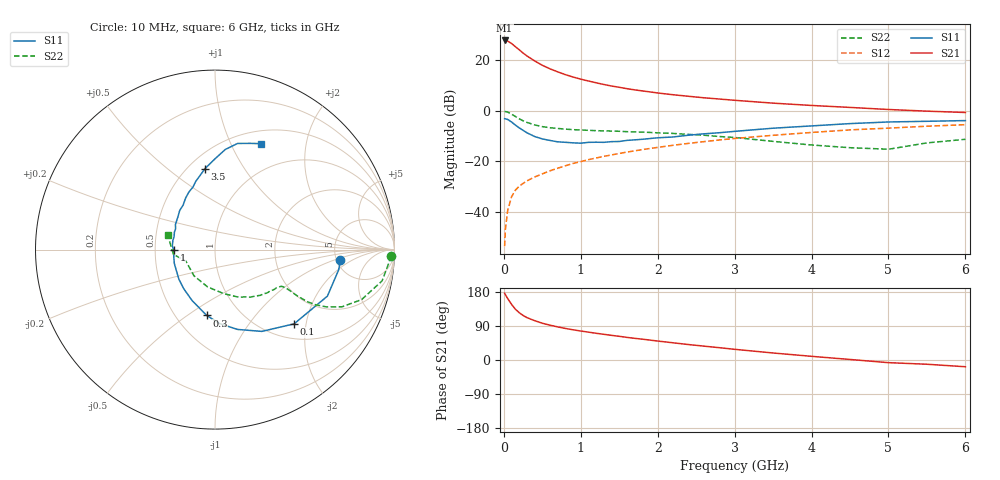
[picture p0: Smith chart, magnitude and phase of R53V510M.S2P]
! SIEMENS Small Signal Semiconductors
! BFR183
! Si NPN RF Bipolar Junction Transistor in SOT23
! VCE = 3.5 V  IC = 10 mA
! Common Emitter S-Parameters:  May  1996
# GHz  S  MA  R  50
!  f  S11  S21  S12  S22
! GHz  MAG  ANG  MAG  ANG  MAG  ANG  MAG  ANG
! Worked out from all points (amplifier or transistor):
!   36 points, 10 MHz to 6 GHz, reference 50 ohm
!   highest |S21| = 27.9 dB at 10 MHz (marker M1)
!   |S21| within 3 dB of that: start of sweep to 172 MHz
!   unconditionally stable (mu >= 1): 774.2 MHz to 2.476 GHz
!   at 250 MHz: K = 0.62, MSG = 25.8 dB, |S12| = -28.7 dB
!   at 1.4 GHz: K = 1.05, MAG = 12.2 dB, |S12| = -17.4 dB
!   at 6 GHz: K = 0.89, MSG = 2.4 dB, |S12| = -5.4 dB
!   lowest NFmin = 1.30 dB at 450 MHz
!   S11 on the Smith chart (normalised r, x): 10 MHz: 5.40, -1.25; 100 MHz: 1.31, -1.71; 300 MHz: 0.70, -0.60; 1 GHz: 0.63, -0.00; 3.5 GHz: 0.60, +0.69; 6 GHz: 0.65, +1.31
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0.01  0.7016 -4.8  24.85 176.3  0.0021 86.6  0.9796 -2.0
0.02  0.6982 -9.3  24.68 172.4  0.0045 86.1  0.972 -4.3
0.05  0.6778 -22.5  24.16 162.1  0.0107 79.8  0.947 -10.6
0.1  0.6044 -43.2  21.63 146.9  0.0199 72.1  0.8633 -18.8
0.15  0.5252 -60.2  18.73 134.0  0.027 66.0  0.7769 -24.2
0.2  0.4623 -74.2  16.25 124.8  0.0323 64.0  0.6988 -27.2
0.25  0.4132 -86.4  14 117.6  0.0367 62.8  0.6369 -28.8
0.3  0.3695 -97.2  12.28 111.9  0.0412 62.8  0.5933 -29.4
0.4  0.3116 -114.1  9.789 103.8  0.0491 62.9  0.5293 -29.4
0.5  0.2792 -128.5  8.017 97.0  0.0567 63.9  0.4884 -28.9
0.6  0.2604 -140.5  6.822 91.9  0.0652 64.6  0.4651 -28.6
0.7  0.2445 -152.0  5.936 87.4  0.0733 65.1  0.4498 -28.5
0.8  0.2393 -161.4  5.228 83.3  0.0821 65.2  0.4365 -28.6
1  0.2297 -179.1  4.259 76.5  0.0992 65.6  0.4195 -29.3
1.1  0.2388 174.6  3.91 73.5  0.1084 65.6  0.4129 -30.3
1.3  0.2388 162.9  3.338 67.8  0.1262 64.8  0.4024 -32.0
1.6  0.2611 147.6  2.759 59.7  0.1531 62.9  0.3885 -35.8
2.2  0.3049 125.6  2.091 45.4  0.2088 58.2  0.3586 -45.3
3.5  0.455 97.0  1.426 18.5  0.3292 43.5  0.2496 -79.0
4.5  0.5611 84.1  1.173 1.4  0.4215 31.3  0.187 -128.9
5.5  0.6233 71.7  0.99 -11.2  0.4982 19.3  0.2329 -173.4
6  0.6441 66.4  0.931 -17.8  0.5343 11.6  0.2744 163.3
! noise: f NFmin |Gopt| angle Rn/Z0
0.45  1.3  0.15  45  0.18
0.9  1.4  0.2  125  0.19
1.8  2.1  0.34  -170  0.14
